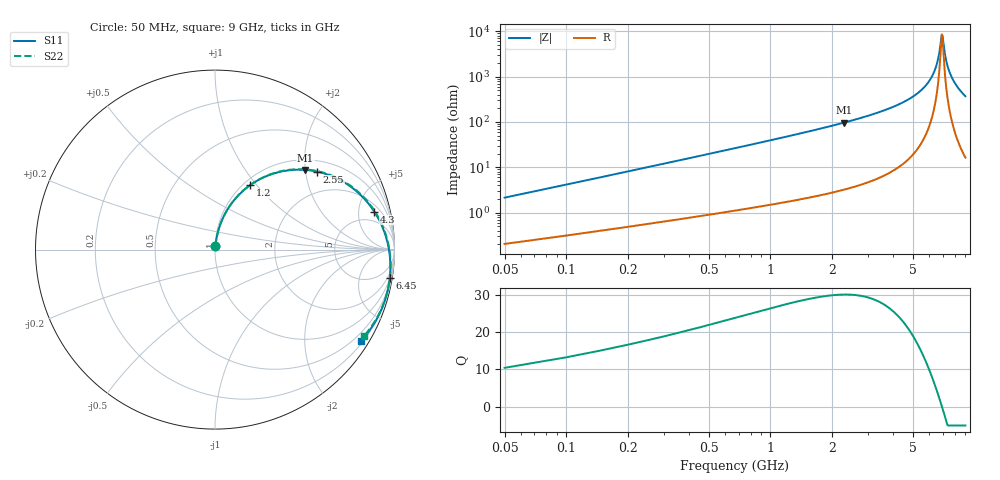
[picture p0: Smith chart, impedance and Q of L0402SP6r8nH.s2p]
!	AVX Thin Film Operation
!	Date:		5 January 2004
!	Description: 	Accu-L®  L0402 Series Thin Film RF Inductors
!	Part Number:	L04026R8BHLTR
!	50 MHz-20GHz Serial Measurements
#	mhz	S	db	R	50
!	S11	S11	S21	S21	S12	S12	S22	S22
!	dB	Phase	dB	Phase	dB	Phase	dB	Phase
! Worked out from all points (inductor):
!   180 points, 50 MHz to 9 GHz, reference 50 ohm
!   read as one part in series: L = 6.6 nH near 50 MHz
!   highest Q = 30 at 2.3 GHz (marker M1), where L = 6.72 nH
!   self-resonance near 6.9 GHz
!   S11 on the Smith chart (normalised r, x): 50 MHz: 1.00, +0.04; 1.2 GHz: 1.07, +0.93; 2.55 GHz: 1.30, +2.32; 4.3 GHz: 2.91, +7.35; 6.45 GHz: 1, -12; 9 GHz: 0.27, -3.47
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50  -33.71 83.0  -0.02 -1.3  -0.02 -1.3  -33.71 83.0
100  -28.00 83.0  -0.03 -2.5  -0.03 -2.5  -28.00 83.0
150  -24.64 82.4  -0.05 -3.6  -0.05 -3.6  -24.64 82.4
350  -17.61 78.7  -0.14 -8.2  -0.14 -8.2  -17.61 78.8
700  -11.94 71.5  -0.39 -16.0  -0.39 -16.0  -11.94 71.6
1200  -7.76 61.3  -0.94 -26.4  -0.94 -26.4  -7.76 61.5
1550  -5.93 54.6  -1.46 -33.2  -1.46 -33.2  -5.93 54.8
2300  -3.46 41.4  -2.88 -46.5  -2.88 -46.5  -3.46 41.7
2550  -2.90 37.3  -3.43 -50.5  -3.43 -50.5  -2.90 37.7
3050  -2.04 29.8  -4.67 -57.9  -4.67 -57.9  -2.04 30.3
4300  -0.80 13.4  -8.58 -73.7  -8.58 -73.7  -0.80 14.1
4550  -0.65 10.5  -9.56 -76.5  -9.56 -76.5  -0.65 11.3
5400  -0.31 1.2  -13.77 -84.6  -13.77 -84.6  -0.31 2.1
6050  -0.16 -5.4  -18.86 -88.6  -18.86 -88.6  -0.17 -4.3
6450  -0.12 -9.2  -24.29 -87.5  -24.29 -87.5  -0.12 -8.1
6700  -0.10 -11.6  -30.55 -78.1  -30.55 -78.1  -0.10 -10.4
6900  -0.10 -13.4  -38.79 -21.9  -38.79 -21.9  -0.10 -12.2
6950  -0.10 -13.9  -38.29 8.5  -38.29 8.5  -0.10 -12.7
7200  -0.10 -16.2  -28.54 57.2  -28.54 57.2  -0.10 -14.9
7550  -0.12 -19.4  -22.03 63.5  -22.03 63.5  -0.12 -17.9
8150  -0.19 -24.6  -16.51 62.1  -16.51 62.1  -0.19 -23.1
9000  -0.36 -31.9  -12.23 56.5  -12.23 56.5  -0.36 -30.1
